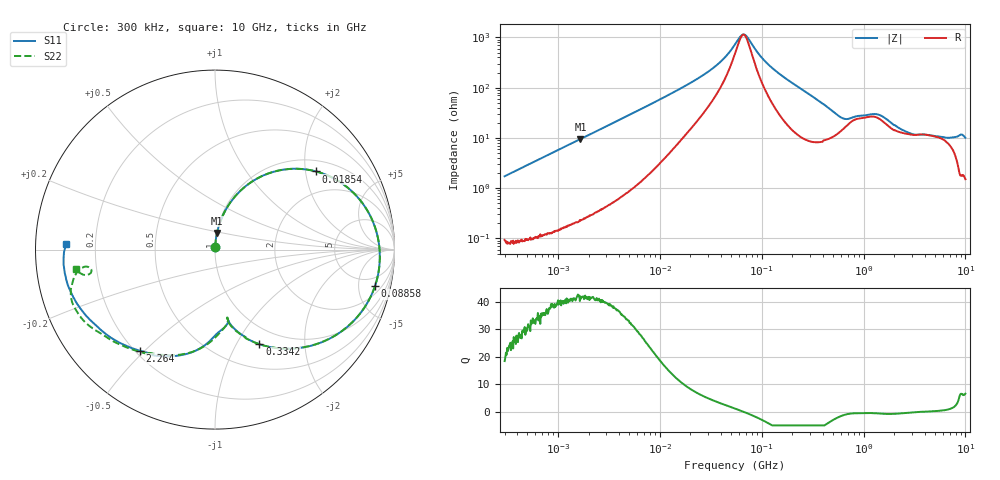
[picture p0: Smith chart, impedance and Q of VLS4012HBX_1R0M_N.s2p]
! S-Parameter Data Generated by TDK Corporation
! Copyright(C) 2023 TDK Corporation.
! All Rights Reserved.
! TDK P/N: VLS4012HBX-1R0M-N (Inductor)
! Property: L=1uH at 1MHz
! Size(LxWxT): 4x4x1.2mm
! Model Type: s2p (Touchstone File Format Version 1.0)
! Frequency: DC=Yes Start=0.3MHz Stop=10000MHz 802points Log-sweep
! Model Generated on June 16, 2023
! Port Assignments:
!  1 ---@@@--- 2
! Applicable Conditions:
!  Temperature = 25 degC
!  DC Bias Current = 0 A
!  Small Signal Operation
! Terms and conditions regarding TDK Simulation Models
! (1)This simulation model is being provided solely for informational purposes. Please refer to the specifications of the products in terms of detailed characteristics of such products.
! (2)In no event shall TDK Corporation of any of its subsidiaries be liable for any loss or damage arising, directly or indirectly,
!  From any information contained in this simulation model, including, but not limited to loss or damages arising from any inaccuracies, omissions or errors in connection with such information.
! (3)Any and all copyrights on this simulation model are owned by TDK Corporation.
!  Duplication or redistribution of this simulation model without prior written permission from TDK Corporation is prohibited.
! (4)This simulation model is subject to any modification or change without any prior notice.
! (5)Neither TDK Corporation nor any of its subsidiaries shall make any warranty, express or implied,
!  Including but not limited to the correctness, implied warranties of merchantability and fitness for a particular purpose with respect to this simulation models.
! (6)The use of this simulation model shall be deemed to have consented to the terms and conditions hereof.
# Hz S MA R 50
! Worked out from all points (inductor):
!   801 points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, 300 kHz to 10 GHz, reference 50 ohm
!   read as one part in series: L = 914 nH near 318.3 kHz
!   highest Q = 41.9 at 1.667 MHz (marker M1), where L = 908 nH
!   self-resonance near 66.24 MHz
!   S11 on the Smith chart (normalised r, x): 300 kHz: 1.00, +0.03; 18.54 MHz: 1.30, +2.29; 88.58 MHz: 3.05, -7.60; 334.2 MHz: 0.78, -1.25; 2.264 GHz: 0.22, -0.48; 10 GHz: 0.09, +0.02
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300000  0.01689 86.0  0.9988 -1.0  0.999 -1.0  0.01679 85.7
1666935  0.09379 83.1  0.9933 -5.5  0.9934 -5.5  0.0938 83.2
1713600  0.09637 83.0  0.9929 -5.6  0.9932 -5.6  0.09641 83.0
4796912  0.2601 73.0  0.9577 -15.3  0.9579 -15.3  0.2601 73.0
9671944  0.4766 58.1  0.8547 -28.9  0.8549 -28.9  0.4766 58.1
1.854358e7  0.7115 37.7  0.6286 -45.9  0.6287 -45.9  0.7115 37.8
3.555278e7  0.8675 16.3  0.3204 -58.6  0.3204 -58.6  0.8675 16.3
5.477226e7  0.9127 2.7  0.1257 -46.1  0.1257 -46.1  0.9129 2.7
6.820897e7  0.92 -4.3  0.08112 6.4  0.08115 6.4  0.9203 -4.2
8.857507e7  0.9141 -13.0  0.1665 50.4  0.1665 50.4  0.9143 -12.9
1.765741e8  0.7984 -39.4  0.5129 43.8  0.5131 43.8  0.7985 -39.3
3.126428e8  0.6057 -62.4  0.7349 21.7  0.7351 21.7  0.605 -62.5
3.342219e8  0.5818 -64.9  0.752 18.9  0.7522 18.9  0.5809 -65.0
5.046115e8  0.4501 -76.6  0.8056 1.8  0.8058 1.8  0.4455 -77.3
7.152593e8  0.4026 -79.3  0.7681 -12.9  0.7683 -12.9  0.3845 -79.6
1.165098e9  0.4943 -91.6  0.6646 -27.4  0.6647 -27.4  0.501 -91.2
1.767019e9  0.6477 -113.3  0.5988 -38.8  0.599 -38.8  0.6513 -115.5
2.264206e9  0.7022 -126.6  0.5598 -48.6  0.56 -48.6  0.71 -126.8
4.632637e9  0.8186 -156.4  0.3521 -79.0  0.3521 -79.0  0.8262 -150.1
6.899057e9  0.8453 -169.2  0.2749 -95.1  0.275 -95.1  0.8425 -162.3
8.322921e9  0.844 -177.3  0.2354 -106.2  0.2355 -106.3  0.7482 -172.2
1e10  0.8322 177.9  0.2232 -110.9  0.2233 -111.0  0.782 -172.2
